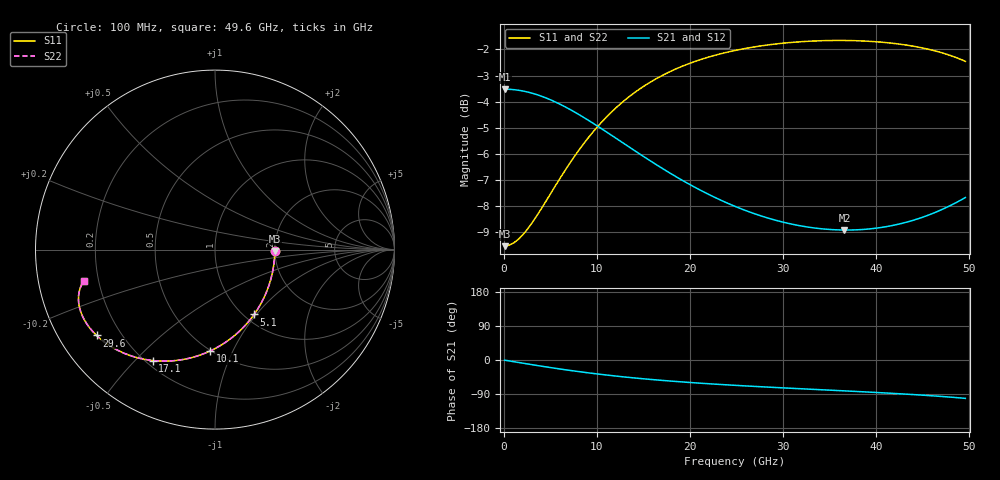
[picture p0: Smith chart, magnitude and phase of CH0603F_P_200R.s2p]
# GHz S RI R 200
! S-Parameters data
! Freq  reS11  imS11  reS21  imS21  reS12  imS12  reS22  imS22
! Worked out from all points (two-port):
!   100 points, 100 MHz to 49.6 GHz, reference 200 ohm
!   highest |S21| = -3.52 dB at 100 MHz (marker M1); lowest = -8.9 dB at 36.6 GHz (marker M2)
!   |S21| within 3 dB of the highest: start of sweep to 16.87 GHz
!   lowest |S11| = -9.5 dB at 100 MHz (marker M3), VSWR 2.00, Z = 400 - j7.02 ohm
!   |S11| at or under -10 dB: nowhere
!   |S22| runs from -9.5 to -1.7 dB; largest |S21 - S12| = 0
!   S11 on the Smith chart (normalised r, x): 100 MHz: 2.00, -0.04; 5.1 GHz: 1.11, -0.97; 10.1 GHz: 0.50, -0.82; 17.1 GHz: 0.23, -0.56; 29.6 GHz: 0.11, -0.32; 49.6 GHz: 0.14, -0.12
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0.1  0.3333 -0.0078  0.6666 -0.00477  0.6666 -0.00477  0.3333 -0.0078
1.1  0.3275 -0.0854  0.663 -0.0522  0.663 -0.0522  0.3275 -0.0854
2.6  0.3012 -0.1976  0.6468 -0.1206  0.6468 -0.1206  0.3012 -0.1976
3.6  0.2731 -0.2674  0.6296 -0.1629  0.6296 -0.1629  0.2731 -0.2674
5.1  0.2178 -0.3616  0.596 -0.2196  0.596 -0.2196  0.2178 -0.3616
6.6  0.1507 -0.4408  0.5558 -0.2669  0.5558 -0.2669  0.1507 -0.4408
8.6  0.0509 -0.5217  0.4971 -0.3148  0.4971 -0.3148  0.0509 -0.5217
10.1  -0.0266 -0.5646  0.4524 -0.3402  0.4524 -0.3402  -0.0266 -0.5646
11.6  -0.103 -0.5941  0.4092 -0.3579  0.4092 -0.3579  -0.103 -0.5941
13.1  -0.1762 -0.6119  0.3685 -0.3694  0.3685 -0.3694  -0.1762 -0.6119
14.6  -0.2449 -0.6203  0.331 -0.376  0.331 -0.376  -0.2449 -0.6203
16.6  -0.3283 -0.6198  0.2862 -0.3793  0.2862 -0.3793  -0.3283 -0.6198
17.1  -0.3476 -0.618  0.276 -0.3794  0.276 -0.3794  -0.3476 -0.618
19.1  -0.4188 -0.6058  0.2384 -0.3778  0.2384 -0.3778  -0.4188 -0.6058
21.1  -0.4807 -0.5874  0.206 -0.3741  0.206 -0.3741  -0.4807 -0.5874
25.1  -0.58 -0.5397  0.1535 -0.3648  0.1535 -0.3648  -0.58 -0.5397
29.6  -0.66 -0.4781  0.1085 -0.3561  0.1085 -0.3561  -0.66 -0.4781
33.1  -0.7041 -0.4282  0.0796 -0.3529  0.0796 -0.3529  -0.7041 -0.4282
36.6  -0.7351 -0.3774  0.0531 -0.354  0.0531 -0.354  -0.7351 -0.3774
41.6  -0.7585 -0.303  0.0139 -0.3645  0.0139 -0.3645  -0.7585 -0.303
46.1  -0.7561 -0.2329  -0.0309 -0.384  -0.0309 -0.384  -0.7561 -0.2329
49.6  -0.7325 -0.1766  -0.0808 -0.4053  -0.0808 -0.4053  -0.7325 -0.1766
